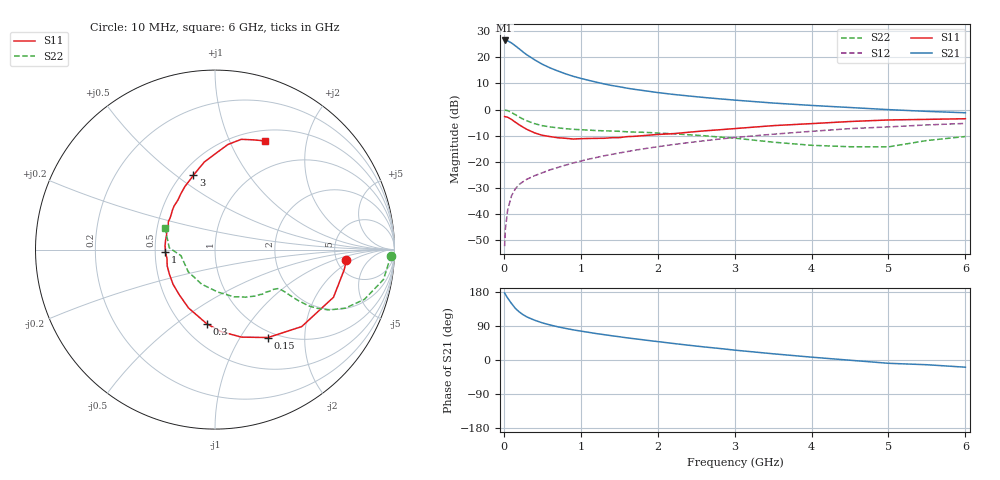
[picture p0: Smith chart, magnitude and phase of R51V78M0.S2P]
! SIEMENS Small Signal Semiconductors
! BFR183
! Si NPN RF Bipolar Junction Transistor in SOT23
! VCE = 1.75 V  IC = 8 mA
! Common Emitter S-Parameters:  May  1996
# GHz  S  MA  R  50
!  f  S11  S21  S12  S22
! GHz  MAG  ANG  MAG  ANG  MAG  ANG  MAG  ANG
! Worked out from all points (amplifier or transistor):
!   36 points, 10 MHz to 6 GHz, reference 50 ohm
!   highest |S21| = 26.5 dB at 10 MHz (marker M1)
!   |S21| within 3 dB of that: start of sweep to 190.6 MHz
!   unconditionally stable (mu >= 1): 810.4 MHz to 2.566 GHz
!   at 250 MHz: K = 0.56, MSG = 24.9 dB, |S12| = -27.7 dB
!   at 1.4 GHz: K = 1.06, MAG = 11.7 dB, |S12| = -17.2 dB
!   at 6 GHz: K = 0.90, MSG = 2.0 dB, |S12| = -5.3 dB
!   S11 on the Smith chart (normalised r, x): 10 MHz: 6.13, -1.57; 150 MHz: 0.91, -1.33; 300 MHz: 0.65, -0.66; 1 GHz: 0.57, -0.02; 3 GHz: 0.57, +0.58; 6 GHz: 0.63, +1.37
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0.01  0.7348 -4.6  21.14 176.8  0.0024 87.2  0.9837 -2.0
0.02  0.7287 -8.8  21.07 173.1  0.0051 86.0  0.9716 -4.1
0.05  0.7116 -21.9  20.8 163.3  0.0119 79.6  0.9532 -10.1
0.1  0.646 -41.6  18.9 149.0  0.0222 72.2  0.8777 -18.4
0.15  0.5721 -58.9  16.66 136.2  0.0303 65.8  0.796 -24.2
0.2  0.5094 -73.2  14.6 127.0  0.0366 62.9  0.7187 -27.9
0.25  0.4589 -85.5  12.68 119.6  0.0414 60.7  0.6552 -29.9
0.3  0.4165 -96.2  11.2 113.6  0.0461 59.7  0.6083 -31.0
0.4  0.3571 -114.4  8.999 105.0  0.054 59.5  0.5363 -31.5
0.5  0.3208 -128.4  7.394 98.0  0.0613 60.3  0.4911 -31.4
0.6  0.3033 -140.4  6.308 92.5  0.0698 60.9  0.4651 -31.2
0.7  0.2882 -152.1  5.508 87.7  0.0774 61.5  0.4461 -31.2
0.8  0.2815 -161.1  4.855 83.5  0.0858 62.0  0.43 -31.3
1  0.2764 -177.1  3.962 76.3  0.1028 62.9  0.4102 -32.0
1.1  0.2789 175.7  3.64 73.1  0.1118 63.0  0.4032 -33.0
1.6  0.3024 149.3  2.574 58.5  0.156 61.0  0.3753 -38.7
2.2  0.3446 126.9  1.955 43.7  0.213 56.7  0.3439 -48.7
3  0.4315 106.2  1.519 26.1  0.2911 48.5  0.2832 -68.2
3.5  0.4914 97.0  1.334 16.4  0.3367 42.2  0.2371 -86.2
4.5  0.5899 83.0  1.094 -0.6  0.4304 29.8  0.1936 -140.5
5.5  0.6485 70.5  0.923 -12.5  0.5072 17.6  0.2549 177.8
6  0.6667 65.2  0.868 -19.0  0.5424 9.7  0.3039 156.4
